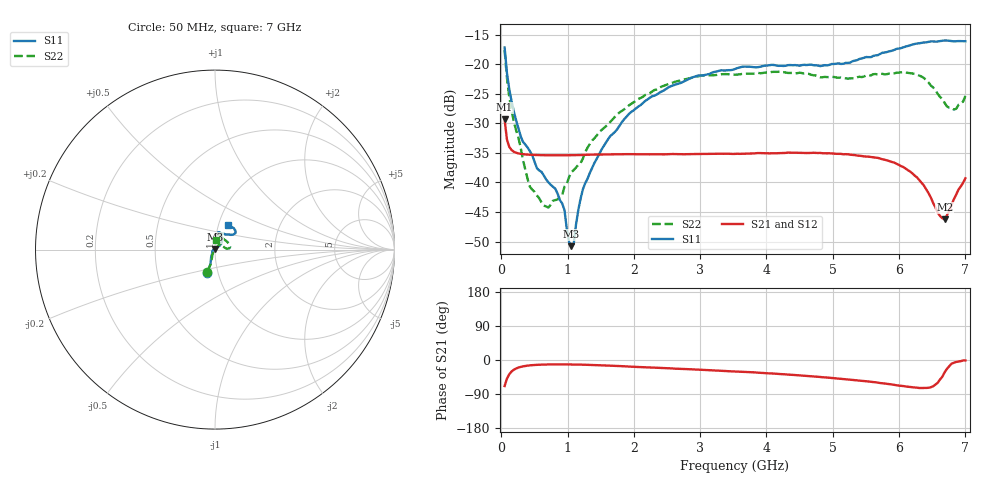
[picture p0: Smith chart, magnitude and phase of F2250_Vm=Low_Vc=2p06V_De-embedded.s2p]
! Integrated Device Technology
! Corporate Headquarters
! 6024 Silver Creek Valley Road
! San Jose, CA 95138  USA
! Phone:  1-408-284-8200
! Toll Free:  1-800-223-1366
! Webpage:  http://www.idt.com/
! Timing and RF Division
! 515 Groton Road, Suite 102
! Westford, MA 01886-6024
! Device:  F2250
! Description: Voltage Variable RF Attenuator
! Frequency:  50.0 -  6000.00 MHz
! Package:  3x3 mm Thin QFN Plastic Package: 16 pin
! Ports:  2 RF, 3 DC
!  Pin  1  = GND
!  Pin  2  = NC
!  Pin  3  = RF1  = Port 1
!  Pin  4  = NC
!  Pin  5  = GND
!  Pin  6  = GND
!  Pin  7  = GND
!  Pin  8  = GND
!  Pin  9  = NC
!  Pin 10  = RF2  = Port 2
!  Pin 11  = NC
!  Pin 12  = GND
!  Pin 13  = GND
!  Pin 14  = VCNTRL
!  Pin 15  = VDD
!  Pin 16  = VMODE
! Vcntrl:  2.060 Volts
! Vmode:  +0.000 Volts
! Vdd:  +3.30  Volts
! Current:  1.180 mA
! Data:  The device was measured on a the F2250 evaluation board which has
!  individual transmission lines to the RF pins.  Data was collected
!  using a calibrated network analyzer.  The evaluation board was
!  de-embedded using a TRL calibration technique.
!  The reference plane is the edge of the package pin.
! Misc:  SN 10
!  Action Tracker AT0258
! Date Measured:  2014-11-26
! Date:  2015-10-15  MJV
! Note:
!  Integrated Device Technology supplies this data as a sample of measured
!  data at the package pin for this product.  Your particular data for this
!  product may vary.
!  Data was taken at 25 degrees C.
!  Integrated Device Technology reserves the right to change this data at anytime.
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# GHz S dB R 50
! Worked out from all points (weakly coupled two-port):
!   201 points, 50 MHz to 7 GHz, reference 50 ohm
!   highest |S21| = -29.32 dB at 50 MHz (marker M1); lowest = -46.3 dB at 6.687 GHz (marker M2)
!   lowest |S11| = -50.8 dB at 1.058 GHz (marker M3), VSWR 1.01, Z = 49.8 + j0.242 ohm
!   |S11| at or under -10 dB: start of sweep to end of sweep
!   |S22| runs from -44.2 to -17.6 dB; largest |S21 - S12| = 6.3e-05
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0.05  -17.18 -108.6  -29.32 -68.7  -29.32 -68.7  -17.64 -109.3
0.08475  -21.44 -107.4  -32.73 -49.4  -32.73 -49.4  -22.27 -105.9
0.189  -28.01 -119.7  -34.81 -25.7  -34.81 -25.8  -29.72 -116.6
0.29325  -32.21 -127.7  -35.17 -18.2  -35.16 -18.2  -34.19 -121.9
0.43225  -34.71 -144.6  -35.31 -14.1  -35.31 -14.1  -40.73 -154.3
0.71025  -39.96 -168.5  -35.40 -11.8  -35.40 -11.8  -44.25 139.0
0.91875  -43.55 158.0  -35.41 -11.6  -35.41 -11.6  -42.13 100.2
0.9535  -44.70 169.9  -35.41 -11.7  -35.41 -11.7  -40.70 102.2
1.023  -50.09 144.1  -35.40 -11.7  -35.41 -11.7  -39.07 84.0
1.05775  -50.77 122.9  -35.40 -11.8  -35.40 -11.8  -38.27 79.9
1.0925  -50.40 89.5  -35.39 -11.9  -35.39 -11.9  -37.91 75.0
1.162  -44.63 56.6  -35.37 -12.1  -35.38 -12.1  -37.01 65.0
1.2315  -41.12 44.0  -35.34 -12.3  -35.34 -12.3  -35.93 57.4
1.6485  -32.11 42.0  -35.26 -15.0  -35.26 -14.9  -29.70 50.6
2.37825  -24.88 47.4  -35.23 -20.7  -35.23 -20.8  -24.08 49.7
3.525  -20.80 72.5  -35.17 -30.2  -35.17 -30.2  -21.76 71.2
4.7065  -20.17 72.4  -34.98 -43.3  -34.98 -43.3  -21.87 70.2
5.85325  -17.82 40.5  -36.39 -63.8  -36.39 -63.8  -21.60 19.2
6.33975  -16.40 41.0  -40.10 -73.9  -40.11 -73.9  -22.10 5.1
6.68725  -15.99 48.8  -46.26 -32.2  -46.24 -31.8  -26.56 25.3
6.861  -16.12 55.1  -42.06 -5.2  -42.02 -5.1  -27.55 58.4
7  -16.12 63.2  -39.30 -1.1  -39.25 -1.3  -25.37 85.9
